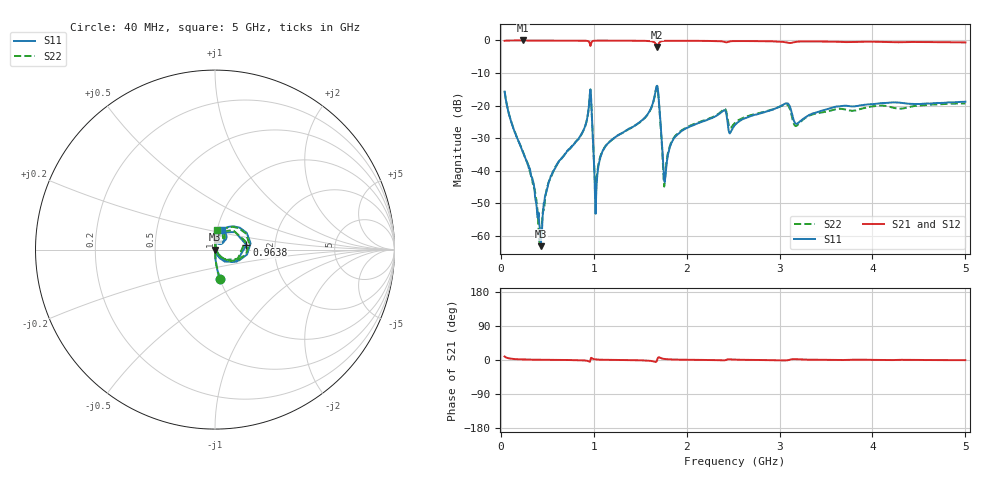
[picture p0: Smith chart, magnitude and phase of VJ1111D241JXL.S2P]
! VJ1111D241JXL
! DATE 02/15/2022  13:29
! CAPACITORS MOUNTED IN SERIES ON 25 MIL THICK MICROSTRIP SUBSTRATE
# GHz  S  MA  R  50.00
!  FREQ  S11M  S11A  S21M  S21A  S12M  S12A  S22M  S22A
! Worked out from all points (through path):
!   801 points, 40 MHz to 5 GHz, reference 50 ohm
!   highest |S21| = 0.00 dB at 238.4 MHz (marker M1); lowest = -2.0 dB at 1.683 GHz (marker M2)
!   lowest |S11| = -63.2 dB at 430.6 MHz (marker M3), VSWR 1.00, Z = 50.1 + j0.00928 ohm
!   |S11| at or under -10 dB: start of sweep to end of sweep
!   |S22| runs from -63.1 to -14.2 dB; largest |S21 - S12| = 0.011
!   S11 on the Smith chart (normalised r, x): 40 MHz: 1.00, -0.33; 963.8 MHz: 1.42, +0.08; 5 GHz: 1.05, +0.23
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0.04  0.1639 -80.2  0.9863 9.3  0.9854 9.5  0.1652 -80.7
0.2384  0.01899 -88.1  0.9998 1.5  0.9987 1.4  0.0194 -88.1
0.3438  0.00708 -80.6  0.9968 0.9  1 0.9  0.006226 -85.5
0.4306  0.0006894 7.7  0.9959 0.6  1.002 0.6  0.001007 40.1
0.536  0.008222 81.5  0.9958 0.4  1 0.4  0.007683 84.1
0.8708  0.03699 83.3  0.9931 -0.6  0.997 -0.8  0.0367 86.7
0.9638  0.177 8.5  0.8228 -0.7  0.8279 -0.7  0.1752 15.4
1.0072  0.00856 -61.1  0.9914 2.0  0.9939 2.0  0.009557 -39.9
1.032  0.006546 75.2  0.9939 1.3  0.9964 1.2  0.007739 61.4
1.1188  0.02293 87.9  0.9948 0.5  0.9975 0.4  0.02307 86.8
1.683  0.2012 10.0  0.7978 0.9  0.8009 0.8  0.1948 10.1
1.6954  0.1472 -24.3  0.8664 7.0  0.8712 7.0  0.1413 -24.2
1.7636  0.006656 28.4  0.9865 2.7  0.9901 2.7  0.006432 46.6
1.8318  0.02573 86.4  0.9892 1.5  0.9949 1.4  0.02688 88.9
1.9434  0.04036 88.1  0.9884 0.8  0.9941 0.7  0.04133 90.3
2.396  0.08386 68.5  0.9588 -0.9  0.9641 -1.0  0.08698 76.0
2.52  0.05029 85.4  0.9786 0.9  0.9845 0.8  0.05403 86.6
3.0656  0.1075 66.5  0.9357 -1.1  0.9424 -1.3  0.1038 70.3
3.1772  0.05237 61.1  0.9536 2.2  0.9583 2.0  0.04839 71.8
3.3508  0.07507 84.2  0.9673 0.7  0.9724 0.5  0.07257 92.4
4.1754  0.1107 74.0  0.9451 -0.2  0.9523 -0.3  0.09597 84.6
5  0.1145 70.3  0.9326 -0.4  0.9386 -0.6  0.1078 83.7
